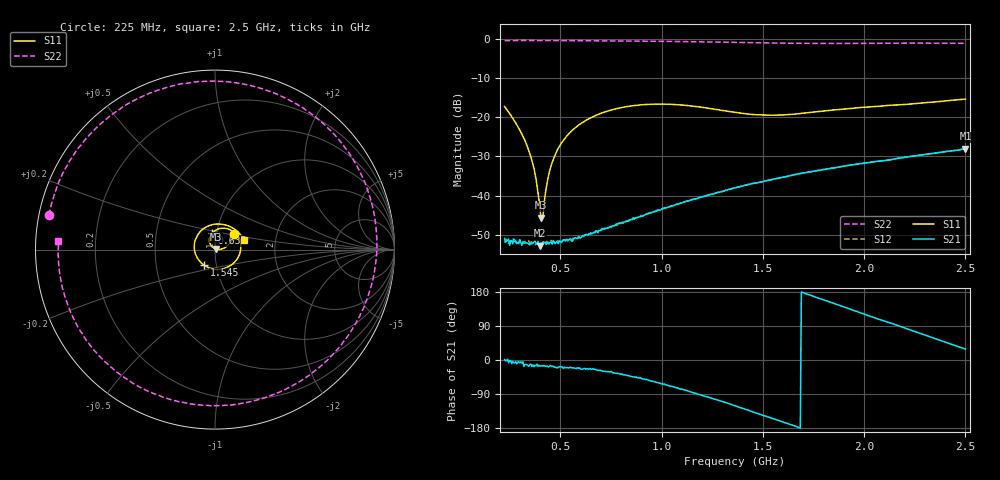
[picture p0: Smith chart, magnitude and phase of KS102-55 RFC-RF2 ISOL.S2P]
!Agilent	"Technologies,E8364B,MY43040668,A.07.50.67"
!Agilent	E8364B:	A.07.50.67
!Date:	"Tuesday,"	September	"22,"	2015	13:34:26
!Correction:	S11(Full	2	"Port(1,2))"
!S21(Full	2	"Port(1,2))"
!S12(Full	2	"Port(1,2))"
!S22(Full	2	"Port(1,2))"
!S2P	File:	Measurements:	"S11,"	"S21,"	"S12,"	S22:
#	Hz	S	dB	R	50
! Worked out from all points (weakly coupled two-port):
!   456 points, 225 MHz to 2.5 GHz, reference 50 ohm
!   highest |S21| = -28.07 dB at 2.5 GHz (marker M1); lowest = -52.8 dB at 400 MHz (marker M2)
!   lowest |S11| = -45.6 dB at 405 MHz (marker M3), VSWR 1.01, Z = 50.3 + j0.404 ohm
!   |S11| at or under -10 dB: start of sweep to end of sweep
!   |S22| runs from -1.2 to -0.5 dB; largest |S21 - S12| = 0.00046
!   S11 on the Smith chart (normalised r, x): 225 MHz: 1.22, +0.21; 635 MHz: 0.95, +0.18; 1.545 GHz: 0.87, -0.15; 2.5 GHz: 1.38, +0.15
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2.25e8  -17.31 38.3  -50.95 1.1  -51.98 2.5  -0.50 168.3
2.95e8  -22.84 16.6  -52.19 -4.5  -52.11 -9.1  -0.46 153.4
3.45e8  -28.59 5.3  -52.40 -16.4  -51.52 -11.1  -0.46 144.1
3.75e8  -34.31 4.4  -51.63 -14.2  -52.65 -16.7  -0.47 138.9
4e8  -43.75 29.6  -52.75 -15.9  -52.41 -15.9  -0.47 134.6
4.05e8  -45.63 50.2  -52.02 -16.0  -52.50 -16.4  -0.47 133.9
4.15e8  -44.88 106.7  -51.75 -16.2  -52.05 -17.8  -0.47 132.1
4.5e8  -33.20 135.2  -51.89 -14.5  -52.09 -17.2  -0.48 126.4
4.8e8  -29.02 133.5  -51.84 -19.3  -52.07 -16.6  -0.48 121.8
5.35e8  -24.66 122.4  -51.17 -20.0  -51.58 -19.8  -0.50 113.3
6.05e8  -21.53 106.7  -50.53 -24.2  -50.24 -21.1  -0.52 102.9
6.35e8  -20.59 99.6  -50.10 -23.8  -50.11 -22.2  -0.54 98.5
8e8  -17.57 63.5  -46.97 -37.5  -47.07 -37.5  -0.59 75.1
9.85e8  -16.68 24.1  -43.77 -60.5  -43.72 -59.9  -0.67 49.4
1.19e9  -17.43 -22.3  -40.39 -91.3  -40.49 -91.6  -0.80 20.0
1.365e9  -18.79 -69.2  -38.02 -121.3  -37.97 -120.7  -0.94 -6.8
1.545e9  -19.51 -124.8  -35.91 -154.2  -35.93 -154.0  -1.10 -36.2
1.745e9  -18.75 176.8  -33.81 169.1  -33.84 168.8  -1.21 -70.0
1.925e9  -17.83 133.7  -32.27 135.4  -32.28 135.3  -1.21 -99.6
2.125e9  -16.99 92.1  -30.93 98.6  -30.87 98.2  -1.17 -130.4
2.305e9  -16.30 57.4  -29.47 64.7  -29.47 65.0  -1.14 -156.3
2.5e9  -15.41 18.1  -28.07 28.7  -28.04 28.7  -1.17 176.9
